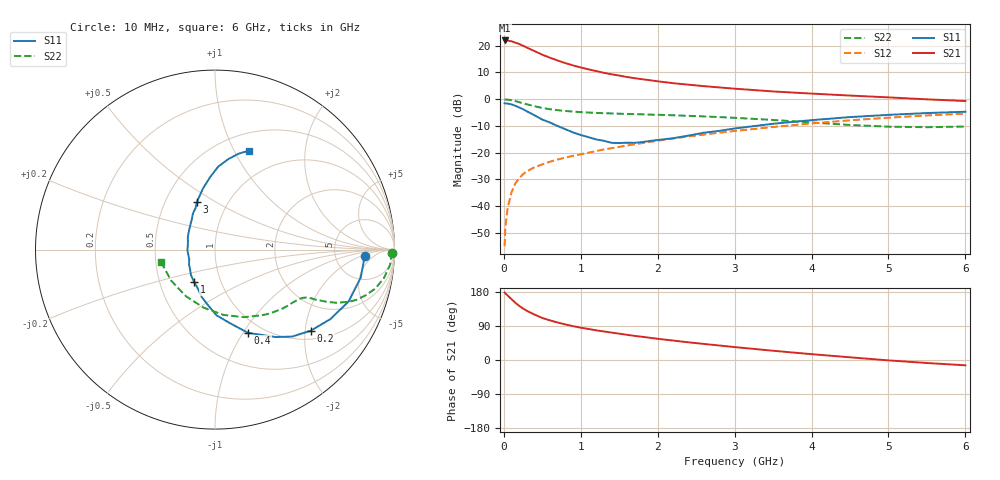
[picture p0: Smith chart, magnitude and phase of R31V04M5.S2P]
! SIEMENS Small Signal Semiconductors
! BFR181
! Si NPN RF Bipolar Junction Transistor in SOT23
! VCE = 1 V  IC = 4.5 mA
! Common Emitter S-Parameters:  May  1996
# GHz  S  MA  R  50
!  f  S11  S21  S12  S22
! GHz  MAG  ANG  MAG  ANG  MAG  ANG  MAG  ANG
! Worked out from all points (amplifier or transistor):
!   36 points, 10 MHz to 6 GHz, reference 50 ohm
!   highest |S21| = 21.9 dB at 10 MHz (marker M1)
!   |S21| within 3 dB of that: start of sweep to 323.5 MHz
!   unconditionally stable (mu >= 1): 986.4 MHz to 3.163 GHz
!   at 250 MHz: K = 0.41, MSG = 24.0 dB, |S12| = -28.0 dB
!   at 1.4 GHz: K = 1.09, MAG = 12.0 dB, |S12| = -18.3 dB
!   at 6 GHz: K = 0.89, MSG = 2.3 dB, |S12| = -5.4 dB
!   S11 on the Smith chart (normalised r, x): 10 MHz: 11, -2; 200 MHz: 1.21, -2.15; 400 MHz: 0.85, -1.05; 1 GHz: 0.75, -0.28; 3 GHz: 0.72, +0.41; 6 GHz: 0.69, +1.15
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0.01  0.8373 -2.3  12.47 178.1  0.0018 93.0  0.9889 -1.0
0.02  0.8319 -4.2  12.26 175.9  0.0041 87.2  0.9826 -2.0
0.05  0.8267 -10.9  12.39 170.0  0.0093 83.6  0.9796 -4.9
0.1  0.7986 -21.2  12.04 160.5  0.0183 79.2  0.9542 -9.6
0.15  0.7508 -31.0  11.33 150.9  0.0268 73.6  0.92 -13.6
0.2  0.6995 -40.2  10.72 142.9  0.0334 69.6  0.8785 -16.8
0.25  0.648 -48.4  9.92 135.8  0.0398 66.8  0.8374 -19.5
0.3  0.5926 -55.3  9.142 129.7  0.045 64.5  0.8007 -21.3
0.4  0.4987 -68.4  7.877 119.7  0.0537 61.8  0.7368 -23.7
0.5  0.4158 -78.9  6.76 110.9  0.0605 60.5  0.6847 -25.1
0.6  0.3664 -88.6  5.932 104.6  0.068 59.9  0.6483 -25.9
0.7  0.3151 -96.6  5.264 98.9  0.0748 59.7  0.6226 -26.5
0.8  0.2745 -105.6  4.706 93.9  0.081 59.7  0.6025 -26.8
1  0.214 -123.2  3.902 85.3  0.0936 60.6  0.5727 -27.8
1.1  0.1951 -133.4  3.604 81.9  0.1002 61.0  0.5624 -28.5
1.6  0.1538 -178.3  2.595 66.5  0.1362 61.5  0.5303 -33.0
2.2  0.1866 139.2  1.988 51.3  0.1842 60.1  0.5002 -40.9
3  0.2834 110.9  1.569 34.1  0.2545 55.4  0.448 -54.8
3.5  0.3473 101.1  1.393 24.4  0.3022 51.2  0.4089 -67.0
4.5  0.4624 87.8  1.167 7.1  0.4027 40.4  0.3296 -101.1
5.5  0.5503 76.2  0.992 -7.9  0.4964 27.3  0.2995 -144.9
6  0.5824 71.1  0.923 -14.0  0.5378 20.1  0.3084 -167.3
